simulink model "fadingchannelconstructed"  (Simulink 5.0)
settings: Solver=ode5  StartTime=0.0  StopTime=10.0  RelTol=1e-3
libraries: commnoisgen2 x2, dspxfrm3 x1, simulink x1

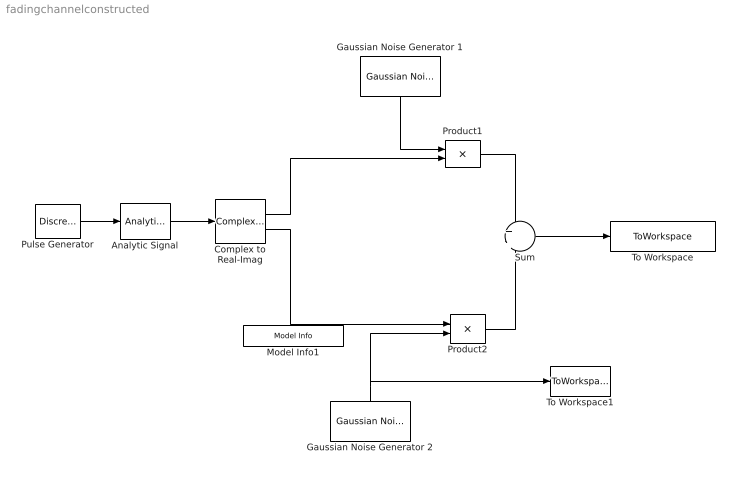
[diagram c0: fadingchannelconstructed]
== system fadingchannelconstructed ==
  Analytic Signal : dspxfrm3/Analytic Signal  N=100
  Complex to Real-Imag : ComplexToRealImag
  Gaussian Noise Generator 1 : commnoisgen2/Gaussian Noise Generator  Orientation=down  m=0  d=0.5  s=41  Ts=.0002  frameBased=off  sampPerFrame=1  orient=on
  Gaussian Noise Generator 2 : commnoisgen2/Gaussian Noise Generator  Orientation=up  m=0  d=0.5  s=41  Ts=.0002  frameBased=off  sampPerFrame=1  orient=off
  Model Info1 : simulink/Model-Wide Utilities/Model Info  InitialBlockCM=None  BlockCM=None  Frame=on  DisplayStringWithTags=Hilbert Transformed  HorizontalTextAlignment=Center  LeftAlignmentValue=0.5  SourceBlockDiagram=fadingchannelconstructed  TagMaxNumber=20
  Product1 : Product  ShowAdditionalParam=on
  Product2 : Product
  Pulse Generator : DiscretePulseGenerator  SampleTime=.0002
  Sum : Sum  Inputs=+|+  ShowAdditionalParam=on
  To Workspace : ToWorkspace  VariableName=RayleighPDFOutput  SampleTime=-1  SaveFormat=Structure
  To Workspace1 : ToWorkspace  VariableName=AWGN  SampleTime=-1  SaveFormat=Structure
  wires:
  Product1/1 -> Sum/1
  Product2/1 -> Sum/2
  Gaussian Noise Generator 1/1 -> Product1/1
  Gaussian Noise Generator 2/1 -> Product2/2, To Workspace1/1
  Sum/1 -> To Workspace/1
  Complex to Real-Imag/1 -> Product1/2
  Complex to Real-Imag/2 -> Product2/1
  Analytic Signal/1 -> Complex to Real-Imag/1
  Pulse Generator/1 -> Analytic Signal/1
